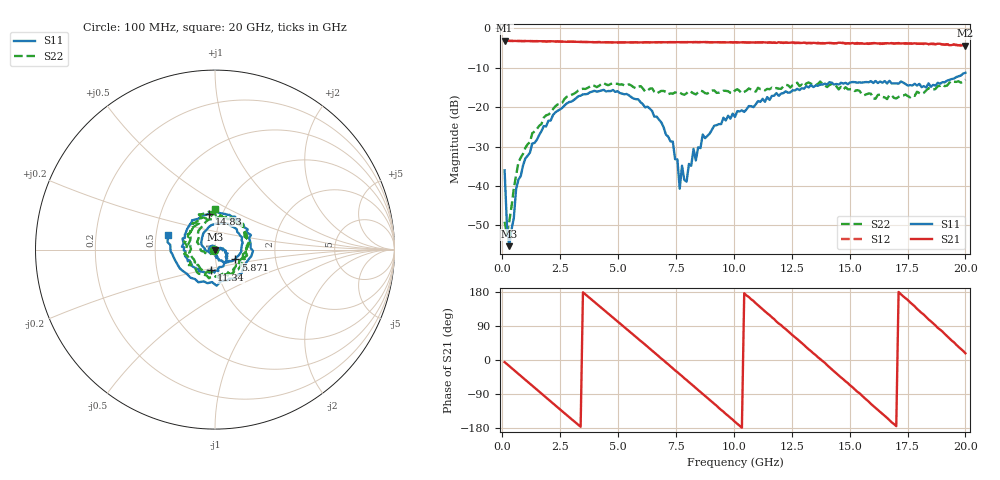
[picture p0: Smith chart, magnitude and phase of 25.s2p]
!Agilent Technologies,N5230C,MY49001569,A.09.33.09
!Agilent N5230C: A.09.33.09
!Date: Thursday, July 23, 2015 14:53:20
!Correction: S11(Full 2 Port(1,2))
!S21(Full 2 Port(1,2))
!S12(Full 2 Port(1,2))
!S22(Full 2 Port(1,2))
!S2P File: Measurements: S11, S21, S12, S22:
# Hz S  dB  R 50
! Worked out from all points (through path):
!   201 points, 100 MHz to 20 GHz, reference 50 ohm
!   highest |S21| = -3.08 dB at 100 MHz (marker M1); lowest = -4.4 dB at 20 GHz (marker M2)
!   group delay of S21, straight-line fit = 147 ps
!   lowest |S11| = -55.2 dB at 299 MHz (marker M3), VSWR 1.00, Z = 49.8 - j0.0341 ohm
!   |S11| at or under -10 dB: start of sweep to end of sweep
!   |S22| runs from -52.2 to -13.0 dB; largest |S21 - S12| = 0.024
!   S11 on the Smith chart (normalised r, x): 100 MHz: 0.97, +0.01; 5.871 GHz: 1.25, -0.14; 11.34 GHz: 0.93, -0.22; 14.83 GHz: 0.87, +0.36; 20 GHz: 0.58, +0.10
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1e8  -36.01 159.4  -3.08 -5.7  -3.06 -5.6  -49.05 -178.6
2.99e8  -55.25 -168.6  -3.17 -16.0  -3.16 -16.0  -49.08 -80.1
5.975e8  -40.70 -106.8  -3.18 -31.6  -3.19 -31.7  -37.28 -115.4
1.294e9  -29.21 -147.7  -3.20 -67.8  -3.24 -67.8  -26.60 -143.3
2.1895e9  -21.97 160.6  -3.27 -114.4  -3.30 -114.4  -20.50 162.7
3.483e9  -16.73 86.4  -3.45 178.6  -3.45 178.7  -15.32 101.1
4.876e9  -16.08 19.3  -3.55 107.1  -3.50 107.1  -14.05 37.4
5.871e9  -18.00 -25.7  -3.58 55.7  -3.57 55.6  -14.79 -3.9
6.7665e9  -23.14 -59.5  -3.50 9.3  -3.49 9.3  -16.17 -31.6
7.3635e9  -28.72 -74.8  -3.49 -22.0  -3.49 -21.7  -16.56 -45.1
7.662e9  -40.67 -65.3  -3.48 -37.5  -3.51 -37.5  -16.28 -49.4
7.7615e9  -34.85 -59.5  -3.51 -42.4  -3.49 -42.6  -16.64 -52.4
7.9605e9  -38.85 -44.2  -3.52 -52.9  -3.47 -53.1  -16.46 -63.6
8.856e9  -27.26 -5.6  -3.46 -100.1  -3.47 -100.2  -16.55 -93.0
1.005e10  -22.46 -33.9  -3.51 -163.2  -3.56 -162.9  -15.74 -149.2
1.13435e10  -18.62 -101.1  -3.57 128.9  -3.63 129.1  -15.71 156.5
1.23385e10  -16.30 -148.2  -3.66 76.2  -3.60 76.2  -14.41 109.6
1.3433e10  -14.87 159.0  -3.66 17.7  -3.77 18.6  -14.20 57.6
1.4826e10  -13.82 99.3  -3.88 -56.4  -3.75 -56.5  -14.93 -20.1
1.67165e10  -13.30 22.1  -3.81 -158.7  -3.86 -159.1  -16.94 -141.8
1.8607e10  -14.33 -102.6  -3.85 96.8  -4.02 96.8  -15.53 144.9
2e10  -11.28 162.7  -4.38 17.8  -4.34 17.6  -12.99 89.3
